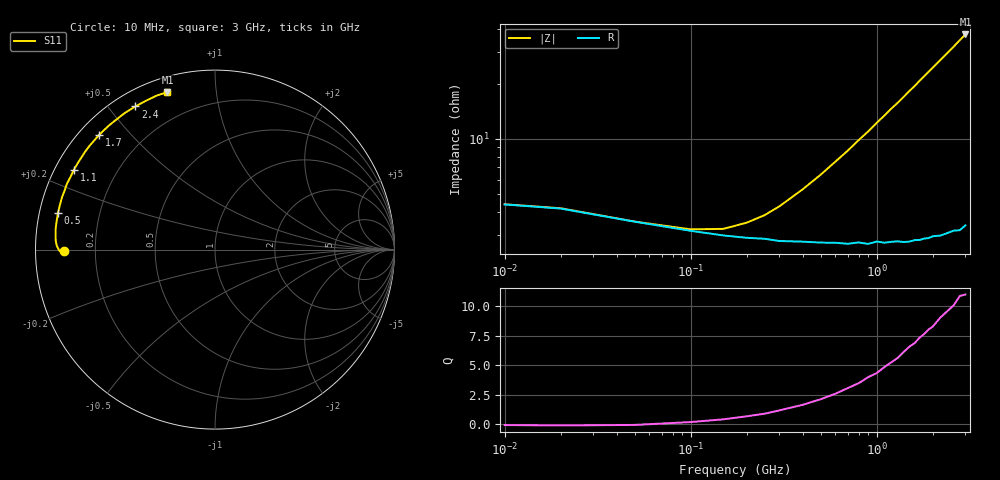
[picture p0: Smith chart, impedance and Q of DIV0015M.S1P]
! SIEMENS Small Signal Semiconductors
! BAV99
! Silicon Switching Diode in SOT23
! IF = 15 mA
! S-Parameters:  May  1995
# GHz  S  MA  R  50
!  f  S11
! GHz  MAG  ANG
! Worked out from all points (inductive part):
!   30 points, 10 MHz to 3 GHz, reference 50 ohm
!   read as one part to ground: L = 1.89 nH near 700 MHz
!   highest Q = 11 at 3 GHz (marker M1), where L = 1.96 nH
!   S11 on the Smith chart (normalised r, x): 10 MHz: 0.09, -0.01; 500 MHz: 0.05, +0.12; 1.1 GHz: 0.05, +0.26; 1.7 GHz: 0.06, +0.41; 2.4 GHz: 0.06, +0.59; 3 GHz: 0.07, +0.74
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0.01  0.8386 -179.4
0.02  0.8462 -179.1
0.05  0.868 -179.6
0.1  0.8815 178.6
0.15  0.8879 177.1
0.2  0.891 175.5
0.25  0.8924 174.1
0.3  0.8954 172.5
0.4  0.8966 169.6
0.5  0.8982 166.8
0.6  0.8991 164.0
0.7  0.9009 161.3
0.8  0.9002 158.5
0.9  0.9028 155.9
1  0.901 153.1
1.1  0.9034 150.5
1.2  0.9036 147.8
1.3  0.9042 145.4
1.4  0.9063 142.8
1.5  0.9072 140.2
1.6  0.9069 137.8
1.7  0.9084 135.2
1.9  0.9095 130.4
2.2  0.9119 123.5
2.4  0.9129 119.1
2.6  0.9141 114.9
2.8  0.9175 110.7
3  0.9166 106.8
